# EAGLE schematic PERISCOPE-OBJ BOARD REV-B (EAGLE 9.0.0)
This Set of Many Schematics Is what comprises the Revision-B PCB, of my eden project "PERISCOPE". (OBJECT BOARD ONLY)

## Sheet 1 of 6: Solder Points For Major Signals
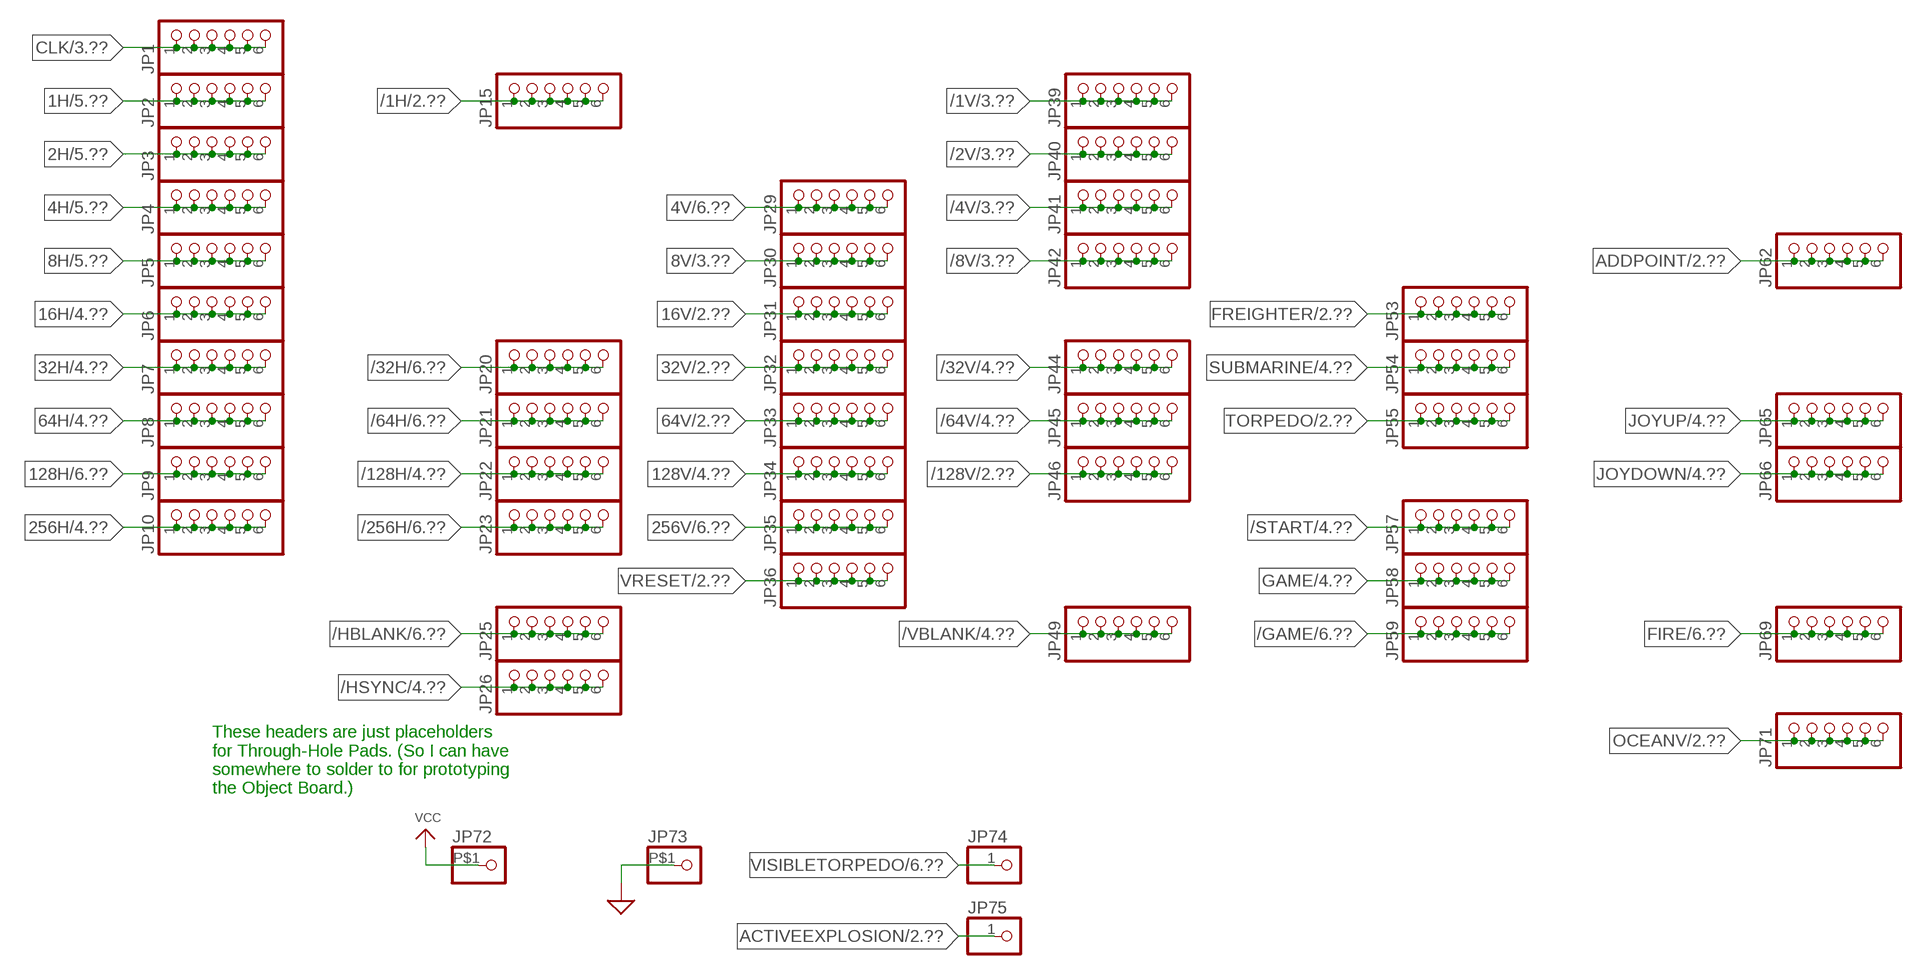
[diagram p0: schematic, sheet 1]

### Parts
JP1  PINHD-1X6  [1X06]
JP2  PINHD-1X6  [1X06]
JP3  PINHD-1X6  [1X06]
JP4  PINHD-1X6  [1X06]
JP5  PINHD-1X6  [1X06]
JP6  PINHD-1X6  [1X06]
JP7  PINHD-1X6  [1X06]
JP8  PINHD-1X6  [1X06]
JP9  PINHD-1X6  [1X06]
JP10  PINHD-1X6  [1X06]
JP15  PINHD-1X6  [1X06]
JP20  PINHD-1X6  [1X06]
JP21  PINHD-1X6  [1X06]
JP22  PINHD-1X6  [1X06]
JP23  PINHD-1X6  [1X06]
JP25  PINHD-1X6  [1X06]
JP26  PINHD-1X6  [1X06]
JP29  PINHD-1X6  [1X06]
JP30  PINHD-1X6  [1X06]
JP31  PINHD-1X6  [1X06]
JP32  PINHD-1X6  [1X06]
JP33  PINHD-1X6  [1X06]
JP34  PINHD-1X6  [1X06]
JP35  PINHD-1X6  [1X06]
JP36  PINHD-1X6  [1X06]
JP39  PINHD-1X6  [1X06]
JP40  PINHD-1X6  [1X06]
JP41  PINHD-1X6  [1X06]
JP42  PINHD-1X6  [1X06]
JP44  PINHD-1X6  [1X06]
JP45  PINHD-1X6  [1X06]
JP46  PINHD-1X6  [1X06]
JP49  PINHD-1X6  [1X06]
JP53  PINHD-1X6  [1X06]
JP54  PINHD-1X6  [1X06]
JP55  PINHD-1X6  [1X06]
JP57  PINHD-1X6  [1X06]
JP58  PINHD-1X6  [1X06]
JP59  PINHD-1X6  [1X06]
JP62  PINHD-1X6  [1X06]
JP65  PINHD-1X6  [1X06]
JP66  PINHD-1X6  [1X06]
JP69  PINHD-1X6  [1X06]
JP71  PINHD-1X6  [1X06]
JP72  PINHD-1X1-BIGPOGO  [1X1-BIGPOGO]
JP73  PINHD-1X1-BIGPOGO  [1X1-BIGPOGO]
JP74  PINHD-1X1  [1X01]
JP75  PINHD-1X1  [1X01]

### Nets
1H: JP2.1 JP2.2 JP2.3 JP2.4 JP2.5 JP2.6 ; also sheet 5
2H: JP3.1 JP3.2 JP3.3 JP3.4 JP3.5 JP3.6 ; also sheet 5
4H: JP4.1 JP4.2 JP4.3 JP4.4 JP4.5 JP4.6 ; also sheet 5
4V: JP29.1 JP29.2 JP29.3 JP29.4 JP29.5 JP29.6 ; also sheet 6
8H: JP5.1 JP5.2 JP5.3 JP5.4 JP5.5 JP5.6 ; also sheet 5,6
8V: JP30.1 JP30.2 JP30.3 JP30.4 JP30.5 JP30.6 ; also sheet 3
16H: JP6.1 JP6.2 JP6.3 JP6.4 JP6.5 JP6.6 ; also sheet 4
16V: JP31.1 JP31.2 JP31.3 JP31.4 JP31.5 JP31.6 ; also sheet 2,4
32H: JP7.1 JP7.2 JP7.3 JP7.4 JP7.5 JP7.6 ; also sheet 4
32V: JP32.1 JP32.2 JP32.3 JP32.4 JP32.5 JP32.6 ; also sheet 2,4
64H: JP8.1 JP8.2 JP8.3 JP8.4 JP8.5 JP8.6 ; also sheet 4
64V: JP33.1 JP33.2 JP33.3 JP33.4 JP33.5 JP33.6 ; also sheet 2,4
128H: JP9.1 JP9.2 JP9.3 JP9.4 JP9.5 JP9.6 ; also sheet 6
128V: JP34.1 JP34.2 JP34.3 JP34.4 JP34.5 JP34.6 ; also sheet 4
256H: JP10.1 JP10.2 JP10.3 JP10.4 JP10.5 JP10.6 ; also sheet 4
256V: JP35.1 JP35.2 JP35.3 JP35.4 JP35.5 JP35.6 ; also sheet 6
/1H: JP15.1 JP15.2 JP15.3 JP15.4 JP15.5 JP15.6 ; also sheet 2
/1V: JP39.1 JP39.2 JP39.3 JP39.4 JP39.5 JP39.6 ; also sheet 3
/2V: JP40.1 JP40.2 JP40.3 JP40.4 JP40.5 JP40.6 ; also sheet 3
/4V: JP41.1 JP41.2 JP41.3 JP41.4 JP41.5 JP41.6 ; also sheet 3
/8V: JP42.1 JP42.2 JP42.3 JP42.4 JP42.5 JP42.6 ; also sheet 3
/32H: JP20.1 JP20.2 JP20.3 JP20.4 JP20.5 JP20.6 ; also sheet 6
/32V: JP44.1 JP44.2 JP44.3 JP44.4 JP44.5 JP44.6 ; also sheet 4
/64H: JP21.1 JP21.2 JP21.3 JP21.4 JP21.5 JP21.6 ; also sheet 6
/64V: JP45.1 JP45.2 JP45.3 JP45.4 JP45.5 JP45.6 ; also sheet 4
/128H: JP22.1 JP22.2 JP22.3 JP22.4 JP22.5 JP22.6 ; also sheet 4
/128V: JP46.1 JP46.2 JP46.3 JP46.4 JP46.5 JP46.6 ; also sheet 2
/256H: JP23.1 JP23.2 JP23.3 JP23.4 JP23.5 JP23.6 ; also sheet 6
/GAME: JP59.1 JP59.2 JP59.3 JP59.4 JP59.5 JP59.6 ; also sheet 6
/HBLANK: JP25.1 JP25.2 JP25.3 JP25.4 JP25.5 JP25.6 ; also sheet 6
/HSYNC: JP26.1 JP26.2 JP26.3 JP26.4 JP26.5 JP26.6 ; also sheet 4,6
/START: JP57.1 JP57.2 JP57.3 JP57.4 JP57.5 JP57.6 ; also sheet 4
/VBLANK: JP49.1 JP49.2 JP49.3 JP49.4 JP49.5 JP49.6 ; also sheet 4,6
ACTIVEEXPLOSION: JP75.1 ; also sheet 2,3
ADDPOINT: JP62.1 JP62.2 JP62.3 JP62.4 JP62.5 JP62.6 ; also sheet 2
CLK: JP1.1 JP1.2 JP1.3 JP1.4 JP1.5 JP1.6 ; also sheet 3,6
FIRE: JP69.1 JP69.2 JP69.3 JP69.4 JP69.5 JP69.6 ; also sheet 6
FREIGHTER: JP53.1 JP53.2 JP53.3 JP53.4 JP53.5 JP53.6 ; also sheet 2
GAME: JP58.1 JP58.2 JP58.3 JP58.4 JP58.5 JP58.6 ; also sheet 4
GND: JP73.P$1 ; supply symbol labelled SUP ; also sheet 2,3,4,5,6
JOYDOWN: JP66.1 JP66.2 JP66.3 JP66.4 JP66.5 JP66.6 ; also sheet 4
JOYUP: JP65.1 JP65.2 JP65.3 JP65.4 JP65.5 JP65.6 ; also sheet 4
OCEANV: JP71.1 JP71.2 JP71.3 JP71.4 JP71.5 JP71.6 ; also sheet 2,6
SUBMARINE: JP54.1 JP54.2 JP54.3 JP54.4 JP54.5 JP54.6 ; also sheet 4
TORPEDO: JP55.1 JP55.2 JP55.3 JP55.4 JP55.5 JP55.6 ; also sheet 2,6
VCC: JP72.P$1 ; also sheet 2,3,4,5,6
VISIBLETORPEDO: JP74.1 ; also sheet 6
VRESET: JP36.1 JP36.2 JP36.3 JP36.4 JP36.5 JP36.6 ; also sheet 2

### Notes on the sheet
- These headers are just placeholders
  for Through-Hole Pads. (So I can have
  somewhere to solder to for prototyping
  the Object Board.)

## Sheet 2 of 6: FREIGHTER MOTION
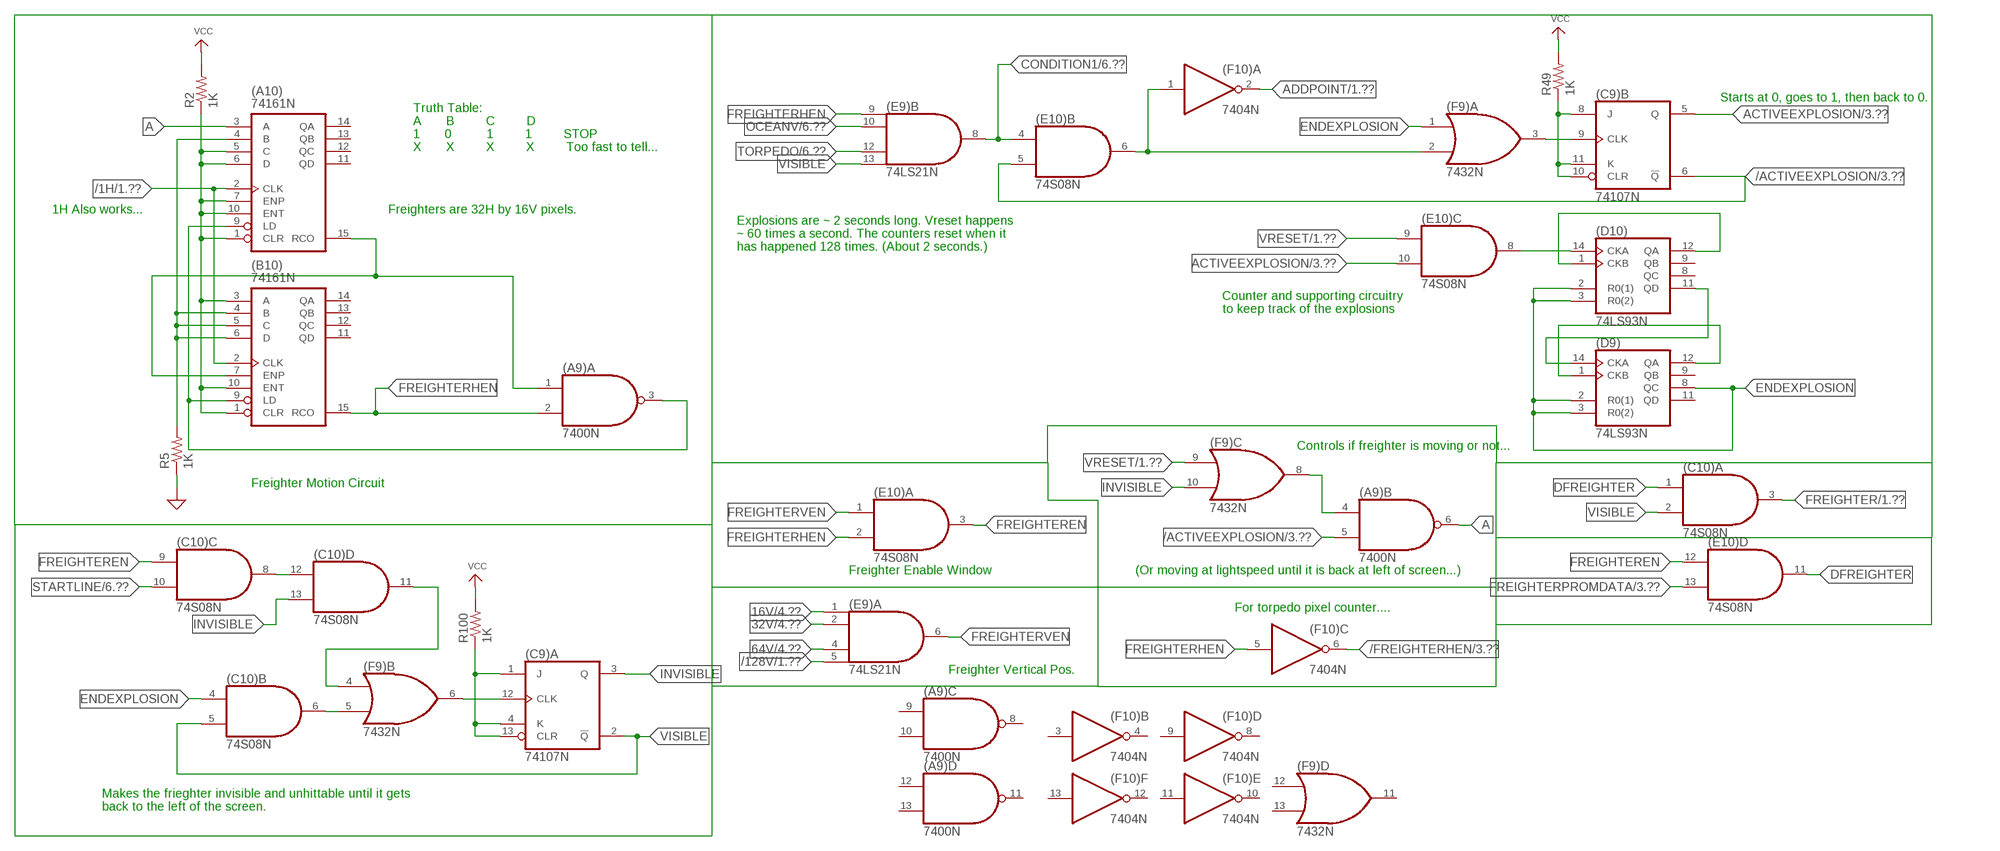
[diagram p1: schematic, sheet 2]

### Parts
(A9)  7400N  [DIL14]
(A10)  74161N  [DIL16]
(B10)  74161N  [DIL16]
(C9)  74107N  [DIL14]
(C10)  74S08N  [DIL14]
(D9)  74LS93N  [DIL14]
(D10)  74LS93N  [DIL14]
(E9)  74LS21N  [DIL14]
(E10)  74S08N  [DIL14]
(F9)  7432N  [DIL14]
(F10)  7404N  [DIL14]
R2  1K  R-US_0207/10  [0207/10]
R5  1K  R-US_0207/10  [0207/10]
R49  1K  R-US_0207/10  [0207/10]
R100  1K  R-US_0207/10  [0207/10]

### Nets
16V: (E9).1(A:I0) ; also sheet 1,4
32V: (E9).2(A:I1) ; also sheet 1,4
64V: (E9).4(A:I2) ; also sheet 1,4
/1H: (A10).2(CLK) (B10).2(CLK) ; also sheet 1
/128V: (E9).5(A:I3) ; also sheet 1
/ACTIVEEXPLOSION: (A9).5(B:I1) (C9).6(B:!Q) (E10).5(B:I1) ; also sheet 3
/FREIGHTERHEN: (F10).6(C:O) ; also sheet 3
A: (A9).6(B:O) (A10).3(A)
ACTIVEEXPLOSION: (C9).5(B:Q) (E10).10(C:I1) ; also sheet 1,3
ADDPOINT: (F10).2(A:O) ; also sheet 1
CONDITION1: (E9).8(B:O) (E10).4(B:I0) ; also sheet 6
DFREIGHTER: (C10).1(A:I0) (E10).11(D:O)
ENDEXPLOSION: (C10).4(B:I0) (D9).2(R0(1)) (D9).3(R0(2)) (D9).8(QC) (D10).2(R0(1)) (D10).3(R0(2)) (F9).1(A:I0)
FREIGHTER: (C10).3(A:O) ; also sheet 1
FREIGHTEREN: (C10).9(C:I0) (E10).3(A:O) (E10).12(D:I0)
FREIGHTERHEN: (A9).2(A:I1) (B10).15(RCO) (E9).9(B:I0) (E10).2(A:I1) (F10).5(C:I)
FREIGHTERPROMDATA: (E10).13(D:I1) ; also sheet 3
FREIGHTERVEN: (E9).6(A:O) (E10).1(A:I0)
GND: R5.1 ; supply symbol labelled SUP ; also sheet 1,3,4,5,6
INVISIBLE: (C9).3(A:Q) (C10).13(D:I1) (F9).10(C:I1)
N$56: (A10).4(B) (B10).4(B) (B10).5(C) (B10).6(D) R5.2
N$57: (A10).1(CLR) (A10).5(C) (A10).6(D) (A10).7(ENP) (A10).10(ENT) (B10).1(CLR) (B10).3(A) (B10).10(ENT) R2.1
N$59: (D10).1(CKB) (D10).12(QA)
N$60: (A9).3(A:O) (A10).9(LD) (B10).9(LD)
N$62: (D9).1(CKB) (D9).12(QA)
N$63: (A9).1(A:I0) (A10).15(RCO) (B10).7(ENP)
N$64: (D10).14(CKA) (E10).8(C:O)
N$67: (D9).14(CKA) (D10).11(QD)
N$68: (C9).9(B:CLK) (F9).3(A:O)
N$69: (C9).8(B:J) (C9).10(B:CLR) (C9).11(B:K) R49.1
N$71: (E10).6(B:O) (F9).2(A:I1) (F10).1(A:I)
N$116: (C9).12(A:CLK) (F9).6(B:O)
N$141: (C10).6(B:O) (F9).5(B:I1)
N$142: (C9).1(A:J) (C9).4(A:K) (C9).13(A:CLR) R100.1
N$143: (C10).8(C:O) (C10).12(D:I0)
N$165: (C10).11(D:O) (F9).4(B:I0)
N$166: (A9).4(B:I0) (F9).8(C:O)
OCEANV: (E9).10(B:I1) ; also sheet 1,6
STARTLINE: (C10).10(C:I1) ; also sheet 6
TORPEDO: (E9).12(B:I2) ; also sheet 1,6
VCC: R2.2 R49.2 R100.2 ; also sheet 1,3,4,5,6
VISIBLE: (C9).2(A:!Q) (C10).2(A:I1) (C10).5(B:I1) (E9).13(B:I3)
VRESET: (E10).9(C:I0) (F9).9(C:I0) ; also sheet 1
Unconnected: (A9).8(C:O) (A9).9(C:I0) (A9).10(C:I1) (A9).11(D:O) (A9).12(D:I0) (A9).13(D:I1) (A10).11(QD) (A10).12(QC) (A10).13(QB) (A10).14(QA) (B10).11(QD) (B10).12(QC) (B10).13(QB) (B10).14(QA) (D9).9(QB) (D9).11(QD) (D10).8(QC) (D10).9(QB) (F9).11(D:O) (F9).12(D:I0) (F9).13(D:I1) (F10).3(B:I) (F10).4(B:O) (F10).8(D:O) (F10).9(D:I) (F10).10(E:O) (F10).11(E:I) (F10).12(F:O) (F10).13(F:I)

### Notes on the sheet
- Starts at 0, goes to 1, then back to 0.
- Truth Table:
  A       B         C         D
  1       0          1         1         STOP
  X       X         X         X         Too fast to tell...
- 1H Also works... | Freighters are 32H by 16V pixels.
- Explosions are ~ 2 seconds long. Vreset happens
  ~ 60 times a second. The counters reset when it
  has happened 128 times. (About 2 seconds.)
- Counter and supporting circuitry
  to keep track of the explosions
- Controls if freighter is moving or not...
- Freighter Motion Circuit
- Freighter Enable Window | (Or moving at lightspeed until it is back at left of screen...)
- For torpedo pixel counter....
- Freighter Vertical Pos.
- Makes the frieghter invisible and unhittable until it gets
  back to the left of the screen.

## Sheet 3 of 6: FREIGHTER GRAPHICS
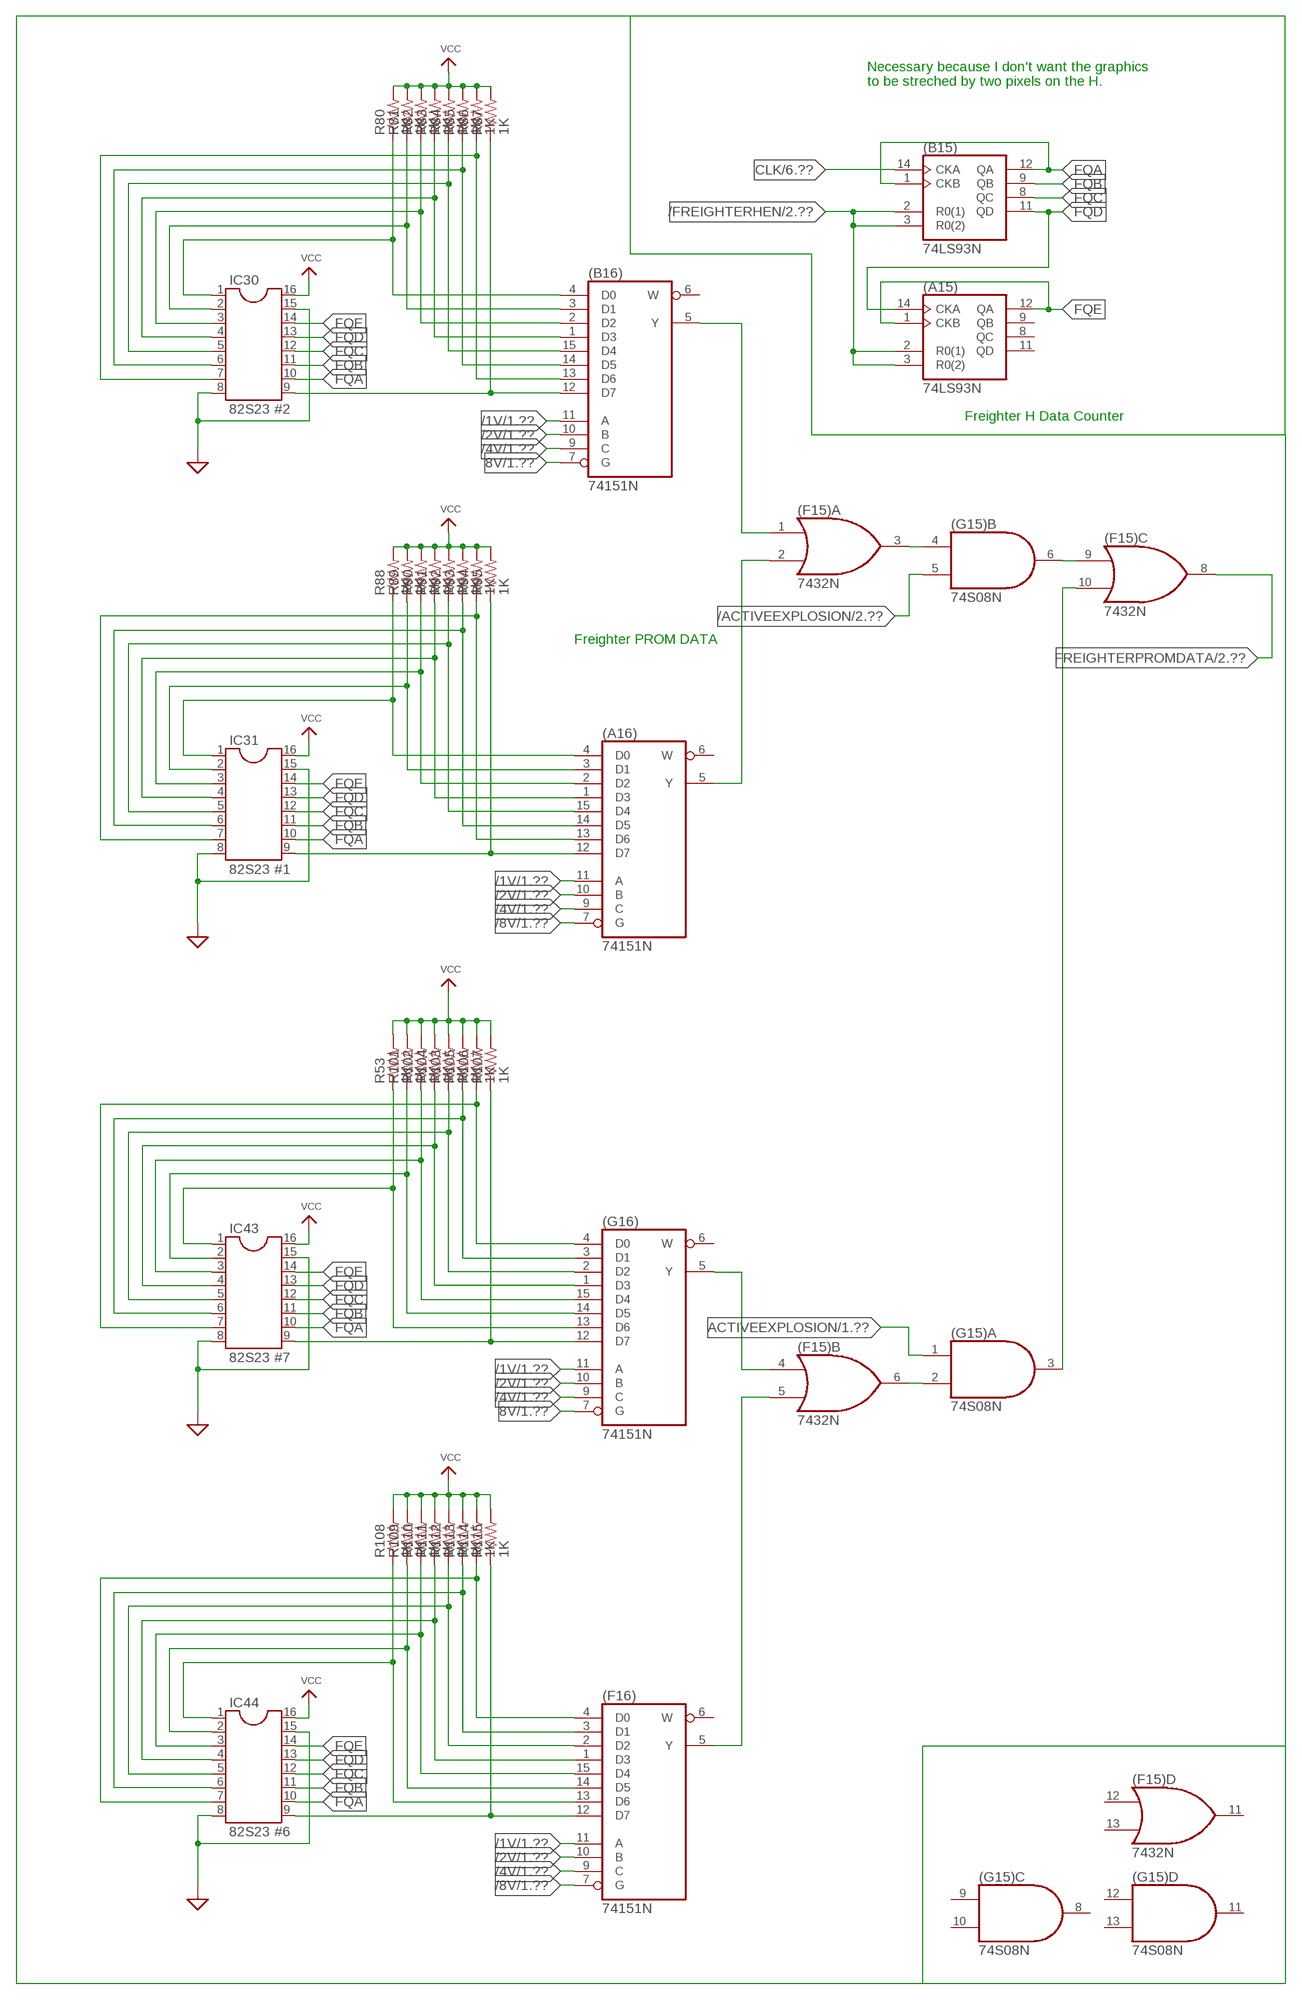
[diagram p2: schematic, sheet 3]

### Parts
(A15)  74LS93N  [DIL14]
(A16)  74151N  [DIL16]
(B15)  74LS93N  [DIL14]
(B16)  74151N  [DIL16]
(F15)  7432N  [DIL14]
(F16)  74151N  [DIL16]
(G15)  74S08N  [DIL14]
(G16)  74151N  [DIL16]
IC30  82S23 #2  DIL16S  [SOCKET-16]
IC31  82S23 #1  DIL16S  [SOCKET-16]
IC43  82S23 #7  DIL16S  [SOCKET-16]
IC44  82S23 #6  DIL16S  [SOCKET-16]
R53  1K  R-US_0207/10  [0207/10]
R80  1K  R-US_0207/10  [0207/10]
R81  1K  R-US_0207/10  [0207/10]
R82  1K  R-US_0207/10  [0207/10]
R83  1K  R-US_0207/10  [0207/10]
R84  1K  R-US_0207/10  [0207/10]
R85  1K  R-US_0207/10  [0207/10]
R86  1K  R-US_0207/10  [0207/10]
R87  1K  R-US_0207/10  [0207/10]
R88  1K  R-US_0207/10  [0207/10]
R89  1K  R-US_0207/10  [0207/10]
R90  1K  R-US_0207/10  [0207/10]
R91  1K  R-US_0207/10  [0207/10]
R92  1K  R-US_0207/10  [0207/10]
R93  1K  R-US_0207/10  [0207/10]
R94  1K  R-US_0207/10  [0207/10]
R95  1K  R-US_0207/10  [0207/10]
R101  1K  R-US_0207/10  [0207/10]
R102  1K  R-US_0207/10  [0207/10]
R103  1K  R-US_0207/10  [0207/10]
R104  1K  R-US_0207/10  [0207/10]
R105  1K  R-US_0207/10  [0207/10]
R106  1K  R-US_0207/10  [0207/10]
R107  1K  R-US_0207/10  [0207/10]
R108  1K  R-US_0207/10  [0207/10]
R109  1K  R-US_0207/10  [0207/10]
R110  1K  R-US_0207/10  [0207/10]
R111  1K  R-US_0207/10  [0207/10]
R112  1K  R-US_0207/10  [0207/10]
R113  1K  R-US_0207/10  [0207/10]
R114  1K  R-US_0207/10  [0207/10]
R115  1K  R-US_0207/10  [0207/10]

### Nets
8V: (B16).7(G) (G16).7(G) ; also sheet 1
/1V: (A16).11(A) (B16).11(A) (F16).11(A) (G16).11(A) ; also sheet 1
/2V: (A16).10(B) (B16).10(B) (F16).10(B) (G16).10(B) ; also sheet 1
/4V: (A16).9(C) (B16).9(C) (F16).9(C) (G16).9(C) ; also sheet 1
/8V: (A16).7(G) (F16).7(G) ; also sheet 1
/ACTIVEEXPLOSION: (G15).5(B:I1) ; also sheet 2
/FREIGHTERHEN: (A15).2(R0(1)) (A15).3(R0(2)) (B15).2(R0(1)) (B15).3(R0(2)) ; also sheet 2
ACTIVEEXPLOSION: (G15).1(A:I0) ; also sheet 1,2
CLK: (B15).14(CKA) ; also sheet 1,6
FQA: (B15).1(CKB) (B15).12(QA) IC30.10 IC31.10 IC43.10 IC44.10
FQB: (B15).9(QB) IC30.11 IC31.11 IC43.11 IC44.11
FQC: (B15).8(QC) IC30.12 IC31.12 IC43.12 IC44.12
FQD: (A15).14(CKA) (B15).11(QD) IC30.13 IC31.13 IC43.13 IC44.13
FQE: (A15).1(CKB) (A15).12(QA) IC30.14 IC31.14 IC43.14 IC44.14
FREIGHTERPROMDATA: (F15).8(C:O) ; also sheet 2
GND: IC30.8 IC30.15 IC31.8 IC31.15 IC43.8 IC43.15 IC44.8 IC44.15 ; supply symbol labelled SUP ; also sheet 1,2,4,5,6
N$58: (F15).3(A:O) (G15).4(B:I0)
N$98: (A16).4(D0) IC31.1 R88.1
N$100: (A16).3(D1) IC31.2 R89.1
N$103: (A16).2(D2) IC31.3 R90.1
N$104: (A16).1(D3) IC31.4 R91.1
N$106: (A16).15(D4) IC31.5 R92.1
N$108: (A16).14(D5) IC31.6 R93.1
N$110: (A16).13(D6) IC31.7 R94.1
N$111: (A16).12(D7) IC31.9 R95.1
N$120: (B16).12(D7) IC30.9 R87.1
N$121: (B16).13(D6) IC30.7 R86.1
N$122: (B16).14(D5) IC30.6 R85.1
N$123: (B16).15(D4) IC30.5 R84.1
N$124: (B16).1(D3) IC30.4 R83.1
N$125: (B16).2(D2) IC30.3 R82.1
N$126: (B16).3(D1) IC30.2 R81.1
N$127: (B16).4(D0) IC30.1 R80.1
N$134: (B16).5(Y) (F15).1(A:I0)
N$135: (A16).5(Y) (F15).2(A:I1)
N$144: (F16).12(D7) IC44.9 R115.1
N$145: (F15).4(B:I0) (G16).5(Y)
N$146: (F15).5(B:I1) (F16).5(Y)
N$147: (F15).9(C:I0) (G15).6(B:O)
N$148: (F15).10(C:I1) (G15).3(A:O)
N$149: (F15).6(B:O) (G15).2(A:I1)
N$150: (G16).12(D7) IC43.9 R107.1
N$151: (G16).13(D6) IC43.1 R53.1
N$152: (G16).14(D5) IC43.2 R101.1
N$153: (G16).15(D4) IC43.3 R102.1
N$154: (G16).1(D3) IC43.4 R104.1
N$155: (G16).2(D2) IC43.5 R103.1
N$156: (G16).3(D1) IC43.6 R105.1
N$157: (G16).4(D0) IC43.7 R106.1
N$158: (F16).13(D6) IC44.1 R108.1
N$159: (F16).14(D5) IC44.2 R109.1
N$160: (F16).15(D4) IC44.3 R110.1
N$161: (F16).1(D3) IC44.4 R111.1
N$162: (F16).2(D2) IC44.5 R112.1
N$163: (F16).3(D1) IC44.6 R113.1
N$164: (F16).4(D0) IC44.7 R114.1
VCC: IC30.16 IC31.16 IC43.16 IC44.16 R53.2 R80.2 R81.2 R82.2 R83.2 R84.2 R85.2 R86.2 R87.2 R88.2 R89.2 R90.2 R91.2 R92.2 R93.2 R94.2 R95.2 R101.2 R102.2 R103.2 R104.2 R105.2 R106.2 R107.2 R108.2 R109.2 R110.2 R111.2 R112.2 R113.2 R114.2 R115.2 ; also sheet 1,2,4,5,6
Unconnected: (A15).8(QC) (A15).9(QB) (A15).11(QD) (A16).6(W) (B16).6(W) (F15).11(D:O) (F15).12(D:I0) (F15).13(D:I1) (F16).6(W) (G15).8(C:O) (G15).9(C:I0) (G15).10(C:I1) (G15).11(D:O) (G15).12(D:I0) (G15).13(D:I1) (G16).6(W)

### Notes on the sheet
- Necessary because I don't want the graphics
  to be streched by two pixels on the H.
- Freighter H Data Counter
- Freighter PROM DATA

## Sheet 4 of 6: SUBMARINE MOTION
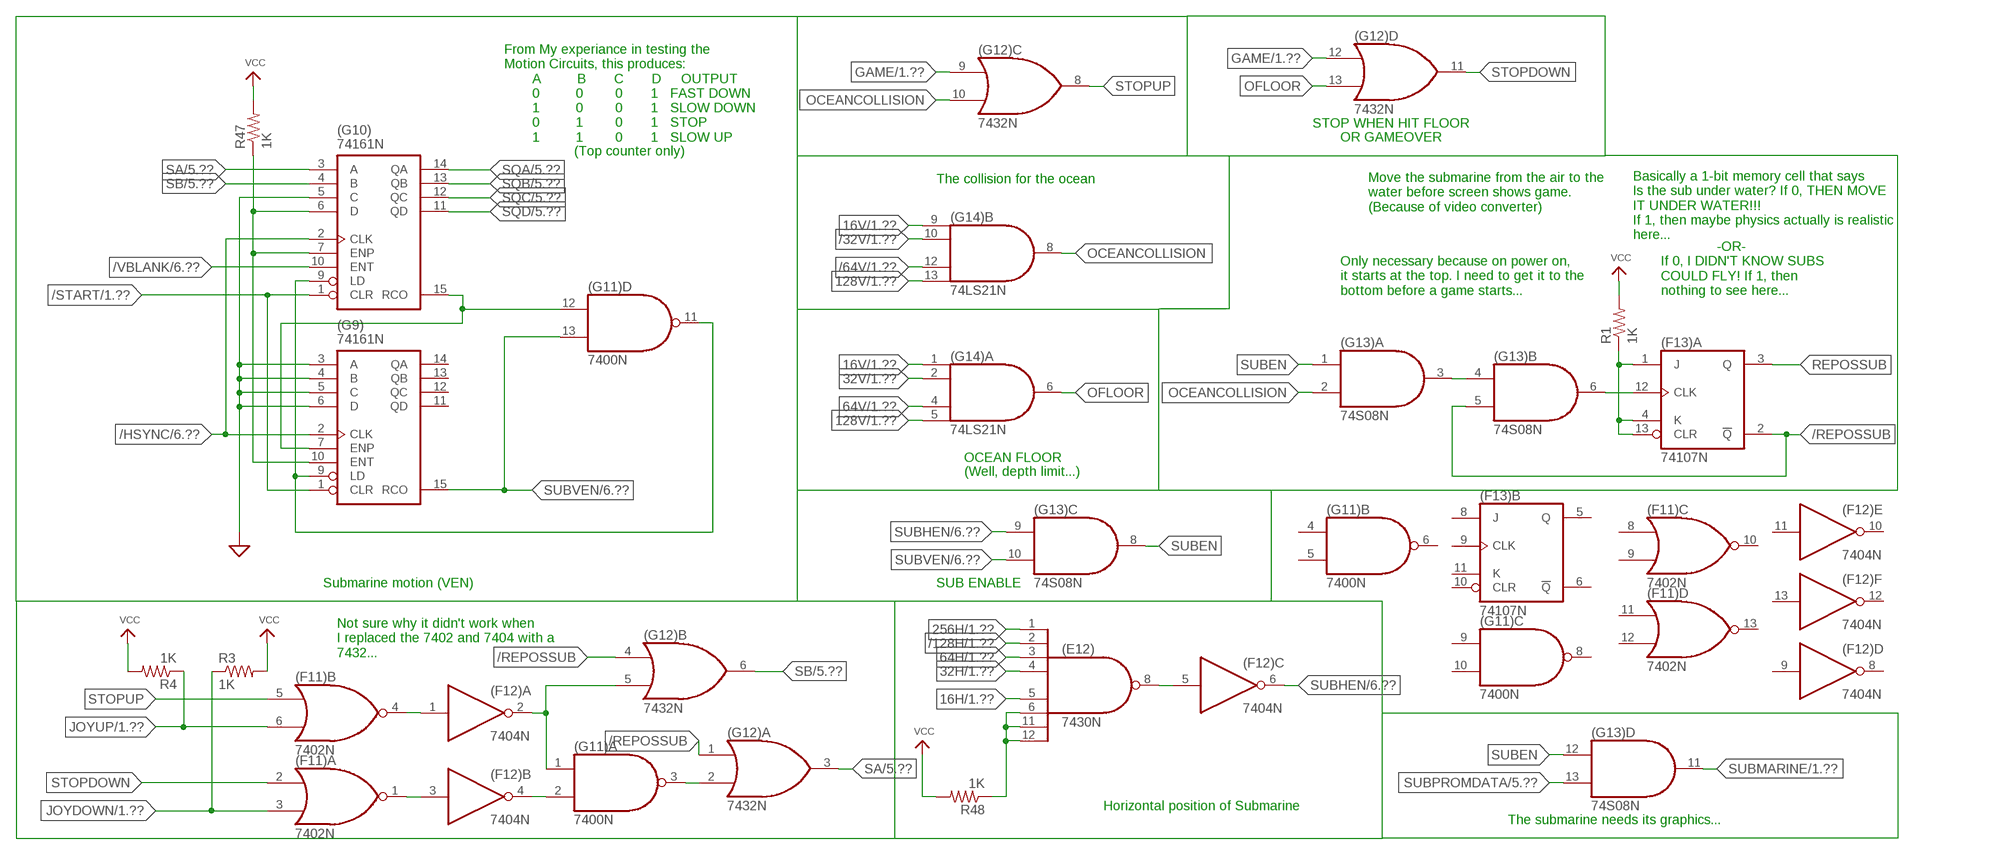
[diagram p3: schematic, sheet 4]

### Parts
(E12)  7430N  [DIL14]
(F11)  7402N  [DIL14]
(F12)  7404N  [DIL14]
(F13)  74107N  [DIL14]
(G9)  74161N  [DIL16]
(G10)  74161N  [DIL16]
(G11)  7400N  [DIL14]
(G12)  7432N  [DIL14]
(G13)  74S08N  [DIL14]
(G14)  74LS21N  [DIL14]
R1  1K  R-US_0207/10  [0207/10]
R3  1K  R-US_0207/10  [0207/10]
R4  1K  R-US_0207/10  [0207/10]
R47  1K  R-US_0207/10  [0207/10]
R48  1K  R-US_0207/10  [0207/10]

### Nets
16H: (E12).5(I4) ; also sheet 1
16V: (G14).1(A:I0) (G14).9(B:I0) ; also sheet 1,2
32H: (E12).4(I3) ; also sheet 1
32V: (G14).2(A:I1) ; also sheet 1,2
64H: (E12).3(I2) ; also sheet 1
64V: (G14).4(A:I2) ; also sheet 1,2
128V: (G14).5(A:I3) (G14).13(B:I3) ; also sheet 1
256H: (E12).1(I0) ; also sheet 1
/32V: (G14).10(B:I1) ; also sheet 1
/64V: (G14).12(B:I2) ; also sheet 1
/128H: (E12).2(I1) ; also sheet 1
/HSYNC: (G9).2(CLK) (G10).2(CLK) ; also sheet 1,6
/REPOSSUB: (F13).2(A:!Q) (G12).1(A:I0) (G12).4(B:I0) (G13).5(B:I1)
/START: (G9).1(CLR) (G10).1(CLR) ; also sheet 1
/VBLANK: (G10).10(ENT) ; also sheet 1,6
BB: (F12).2(A:O) (G11).1(A:I0) (G12).5(B:I1)
GAME: (G12).9(C:I0) (G12).12(D:I0) ; also sheet 1
GND: (G9).3(A) (G9).4(B) (G9).5(C) (G9).6(D) (G10).5(C) ; supply symbol labelled SUP ; also sheet 1,2,3,5,6
JOYDOWN: (F11).3(A:I1) R3.1 ; also sheet 1
JOYUP: (F11).6(B:I1) R4.1 ; also sheet 1
N$1: (F11).1(A:O) (F12).3(B:I)
N$9: (F12).4(B:O) (G11).2(A:I1)
N$41: (F11).4(B:O) (F12).1(A:I)
N$48: (E12).8(O) (F12).5(C:I)
N$50: (G9).10(ENT) (G10).6(D) (G10).7(ENP) R47.1
N$51: (G9).9(LD) (G10).9(LD) (G11).11(D:O)
N$52: (E12).6(I5) (E12).11(I6) (E12).12(I7) R48.1
N$53: (F13).1(A:J) (F13).4(A:K) (F13).13(A:CLR) R1.1
N$54: (G13).3(A:O) (G13).4(B:I0)
N$55: (F13).12(A:CLK) (G13).6(B:O)
N$170: (G11).3(A:O) (G12).2(A:I1)
N$173: (G9).7(ENP) (G10).15(RCO) (G11).12(D:I0)
OCEANCOLLISION: (G12).10(C:I1) (G13).2(A:I1) (G14).8(B:O)
OFLOOR: (G12).13(D:I1) (G14).6(A:O)
REPOSSUB: (F13).3(A:Q)
SA: (G10).3(A) (G12).3(A:O) ; also sheet 5,6
SB: (G10).4(B) (G12).6(B:O) ; also sheet 5,6
SQA: (G10).14(QA) ; also sheet 5
SQB: (G10).13(QB) ; also sheet 5,6
SQC: (G10).12(QC) ; also sheet 5
SQD: (G10).11(QD) ; also sheet 5,6
STOPDOWN: (F11).2(A:I0) (G12).11(D:O)
STOPUP: (F11).5(B:I0) (G12).8(C:O)
SUBEN: (G13).1(A:I0) (G13).8(C:O) (G13).12(D:I0)
SUBHEN: (F12).6(C:O) (G13).9(C:I0) ; also sheet 6
SUBMARINE: (G13).11(D:O) ; also sheet 1
SUBPROMDATA: (G13).13(D:I1) ; also sheet 5
SUBVEN: (G9).15(RCO) (G11).13(D:I1) (G13).10(C:I1) ; also sheet 6
VCC: R1.2 R3.2 R4.2 R47.2 R48.2 ; also sheet 1,2,3,5,6
Unconnected: (F11).8(C:I0) (F11).9(C:I1) (F11).10(C:O) (F11).11(D:I0) (F11).12(D:I1) (F11).13(D:O) (F12).8(D:O) (F12).9(D:I) (F12).10(E:O) (F12).11(E:I) (F12).12(F:O) (F12).13(F:I) (F13).5(B:Q) (F13).6(B:!Q) (F13).8(B:J) (F13).9(B:CLK) (F13).10(B:CLR) (F13).11(B:K) (G9).11(QD) (G9).12(QC) (G9).13(QB) (G9).14(QA) (G11).4(B:I0) (G11).5(B:I1) (G11).6(B:O) (G11).8(C:O) (G11).9(C:I0) (G11).10(C:I1)

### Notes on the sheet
- STOP WHEN HIT FLOOR
- From My experiance in testing the 
  Motion Circuits, this produces:
         A         B       C       D     OUTPUT
         0         0        0       1   FAST DOWN
         1         0        0       1   SLOW DOWN
         0         1        0       1   STOP
         1         1        0       1   SLOW UP
- OR GAMEOVER
- (Top counter only)
- The collision for the ocean
- Move the submarine from the air to the
  water before screen shows game. 
  (Because of video converter)
- Basically a 1-bit memory cell that says
  Is the sub under water? If 0, THEN MOVE
  IT UNDER WATER!!!
  If 1, then maybe physics actually is realistic
  here...
- Only necessary because on power on,
  it starts at the top. I need to get it to the
  bottom before a game starts...
- -OR-
  If 0, I DIDN'T KNOW SUBS
  COULD FLY! If 1, then 
  nothing to see here...
- OCEAN FLOOR
- (Well, depth limit...)
- Submarine motion (VEN) | SUB ENABLE
- Not sure why it didn't work when
  I replaced the 7402 and 7404 with a
  7432...
- Horizontal position of Submarine
- The submarine needs its graphics...

## Sheet 5 of 6: SUBMARINE GRAPHICS
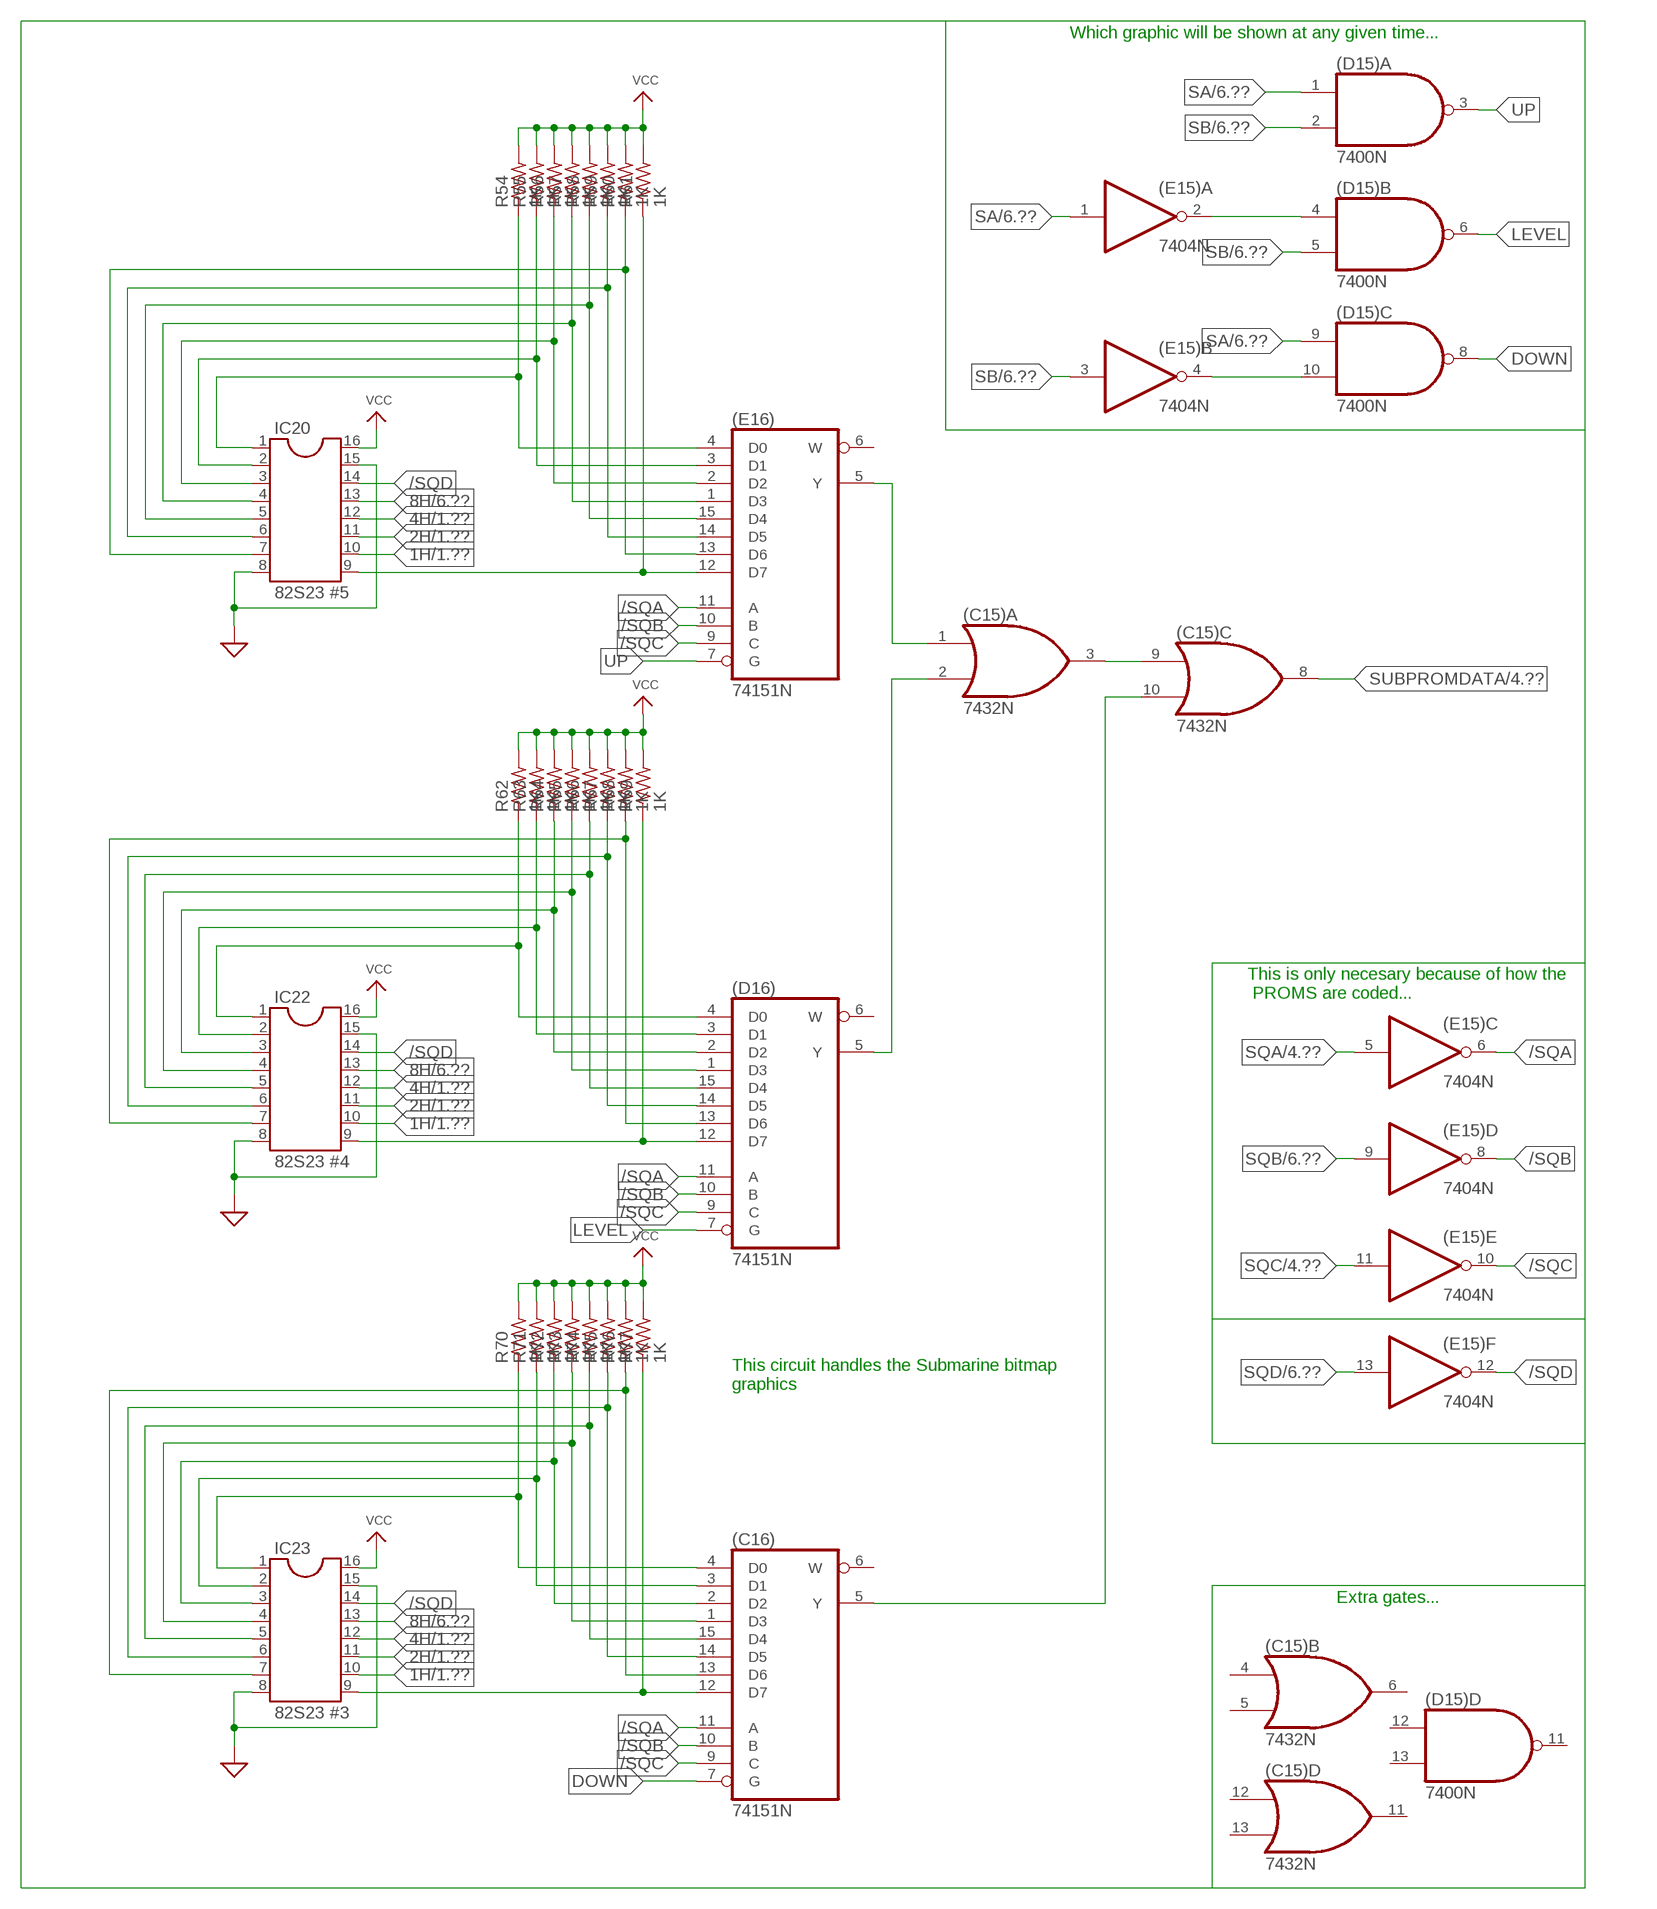
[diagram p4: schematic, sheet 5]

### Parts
(C15)  7432N  [DIL14]
(C16)  74151N  [DIL16]
(D15)  7400N  [DIL14]
(D16)  74151N  [DIL16]
(E15)  7404N  [DIL14]
(E16)  74151N  [DIL16]
IC20  82S23 #5  DIL16S  [SOCKET-16]
IC22  82S23 #4  DIL16S  [SOCKET-16]
IC23  82S23 #3  DIL16S  [SOCKET-16]
R54  1K  R-US_0207/10  [0207/10]
R55  1K  R-US_0207/10  [0207/10]
R56  1K  R-US_0207/10  [0207/10]
R57  1K  R-US_0207/10  [0207/10]
R58  1K  R-US_0207/10  [0207/10]
R59  1K  R-US_0207/10  [0207/10]
R60  1K  R-US_0207/10  [0207/10]
R61  1K  R-US_0207/10  [0207/10]
R62  1K  R-US_0207/10  [0207/10]
R63  1K  R-US_0207/10  [0207/10]
R64  1K  R-US_0207/10  [0207/10]
R65  1K  R-US_0207/10  [0207/10]
R66  1K  R-US_0207/10  [0207/10]
R67  1K  R-US_0207/10  [0207/10]
R68  1K  R-US_0207/10  [0207/10]
R69  1K  R-US_0207/10  [0207/10]
R70  1K  R-US_0207/10  [0207/10]
R71  1K  R-US_0207/10  [0207/10]
R72  1K  R-US_0207/10  [0207/10]
R73  1K  R-US_0207/10  [0207/10]
R74  1K  R-US_0207/10  [0207/10]
R75  1K  R-US_0207/10  [0207/10]
R76  1K  R-US_0207/10  [0207/10]
R77  1K  R-US_0207/10  [0207/10]

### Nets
1H: IC20.10 IC22.10 IC23.10 ; also sheet 1
2H: IC20.11 IC22.11 IC23.11 ; also sheet 1
4H: IC20.12 IC22.12 IC23.12 ; also sheet 1
8H: IC20.13 IC22.13 IC23.13 ; also sheet 1,6
/SQA: (C16).11(A) (D16).11(A) (E15).6(C:O) (E16).11(A)
/SQB: (C16).10(B) (D16).10(B) (E15).8(D:O) (E16).10(B)
/SQC: (C16).9(C) (D16).9(C) (E15).10(E:O) (E16).9(C)
/SQD: (E15).12(F:O) IC20.14 IC22.14 IC23.14
DOWN: (C16).7(G) (D15).8(C:O)
GND: IC20.8 IC20.15 IC22.8 IC22.15 IC23.8 IC23.15 ; supply symbol labelled SUP ; also sheet 1,2,3,4,6
LEVEL: (D15).6(B:O) (D16).7(G)
N$65: (C15).1(A:I0) (E16).5(Y)
N$66: (C15).2(A:I1) (D16).5(Y)
N$72: (C15).10(C:I1) (C16).5(Y)
N$73: (E16).12(D7) IC20.9 R61.1
N$74: (E16).1(D3) IC20.4 R57.1
N$75: (E16).15(D4) IC20.5 R58.1
N$76: (C15).3(A:O) (C15).9(C:I0)
N$77: (E16).14(D5) IC20.6 R59.1
N$78: (E16).13(D6) IC20.7 R60.1
N$79: (C16).4(D0) IC23.1 R70.1
N$80: (D16).4(D0) IC22.1 R62.1
N$81: (D16).3(D1) IC22.2 R63.1
N$82: (D16).12(D7) IC22.9 R69.1
N$83: (C16).12(D7) IC23.9 R77.1
N$84: (E16).4(D0) IC20.1 R54.1
N$85: (E16).3(D1) IC20.2 R55.1
N$86: (E16).2(D2) IC20.3 R56.1
N$87: (D16).2(D2) IC22.3 R64.1
N$88: (D16).1(D3) IC22.4 R65.1
N$89: (D16).15(D4) IC22.5 R66.1
N$90: (D16).14(D5) IC22.6 R67.1
N$91: (D16).13(D6) IC22.7 R68.1
N$92: (C16).3(D1) IC23.2 R71.1
N$93: (C16).2(D2) IC23.3 R72.1
N$94: (C16).1(D3) IC23.4 R73.1
N$95: (C16).15(D4) IC23.5 R74.1
N$96: (C16).14(D5) IC23.6 R75.1
N$97: (C16).13(D6) IC23.7 R76.1
N$102: (D15).10(C:I1) (E15).4(B:O)
N$105: (D15).4(B:I0) (E15).2(A:O)
SA: (D15).1(A:I0) (D15).9(C:I0) (E15).1(A:I) ; also sheet 4,6
SB: (D15).2(A:I1) (D15).5(B:I1) (E15).3(B:I) ; also sheet 4,6
SQA: (E15).5(C:I) ; also sheet 4
SQB: (E15).9(D:I) ; also sheet 4,6
SQC: (E15).11(E:I) ; also sheet 4
SQD: (E15).13(F:I) ; also sheet 4,6
SUBPROMDATA: (C15).8(C:O) ; also sheet 4
UP: (D15).3(A:O) (E16).7(G)
VCC: IC20.16 IC22.16 IC23.16 R54.2 R55.2 R56.2 R57.2 R58.2 R59.2 R60.2 R61.2 R62.2 R63.2 R64.2 R65.2 R66.2 R67.2 R68.2 R69.2 R70.2 R71.2 R72.2 R73.2 R74.2 R75.2 R76.2 R77.2 ; also sheet 1,2,3,4,6
Unconnected: (C15).4(B:I0) (C15).5(B:I1) (C15).6(B:O) (C15).11(D:O) (C15).12(D:I0) (C15).13(D:I1) (C16).6(W) (D15).11(D:O) (D15).12(D:I0) (D15).13(D:I1) (D16).6(W) (E16).6(W)

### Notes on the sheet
- Which graphic will be shown at any given time...
- This is only necesary because of how the
   PROMS are coded...
- This circuit handles the Submarine bitmap
  graphics
- Extra gates...

## Sheet 6 of 6: TORPEDO MOTION
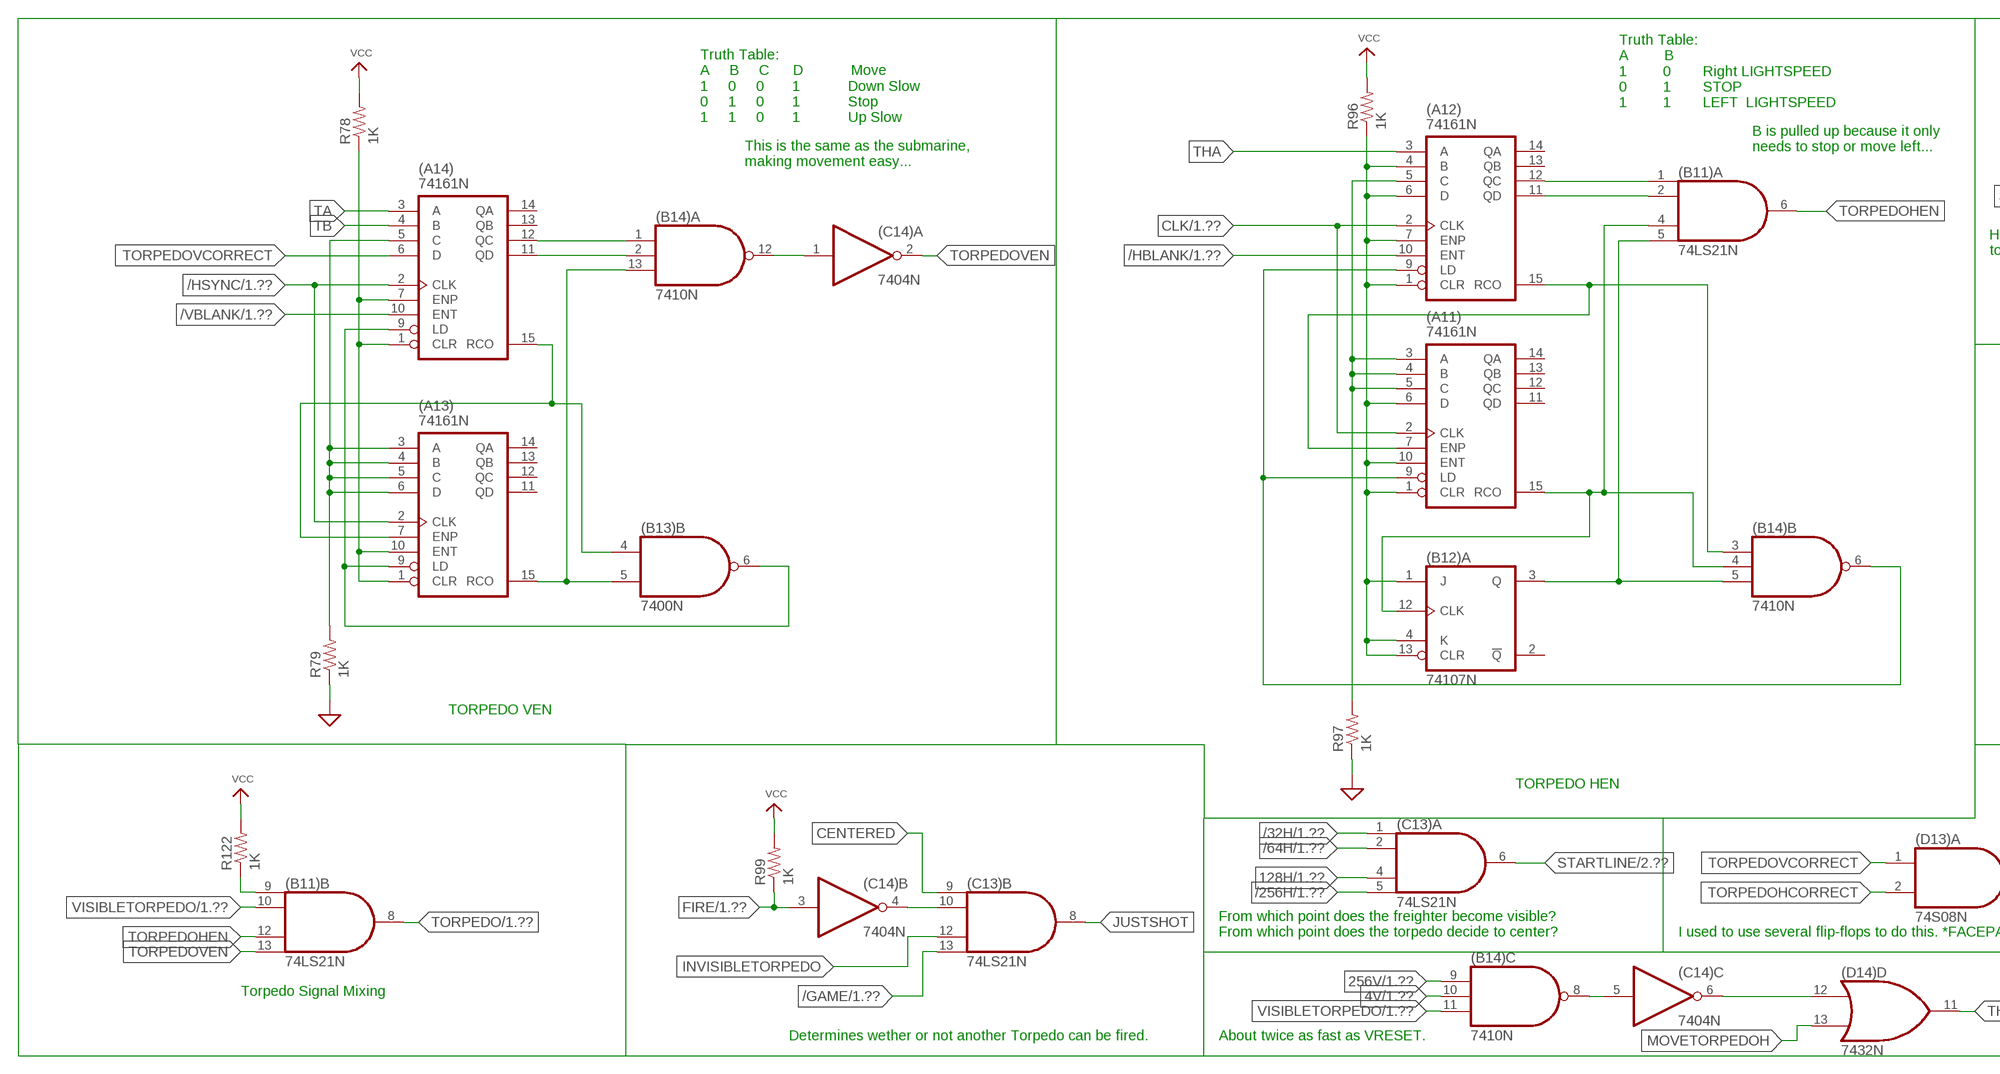
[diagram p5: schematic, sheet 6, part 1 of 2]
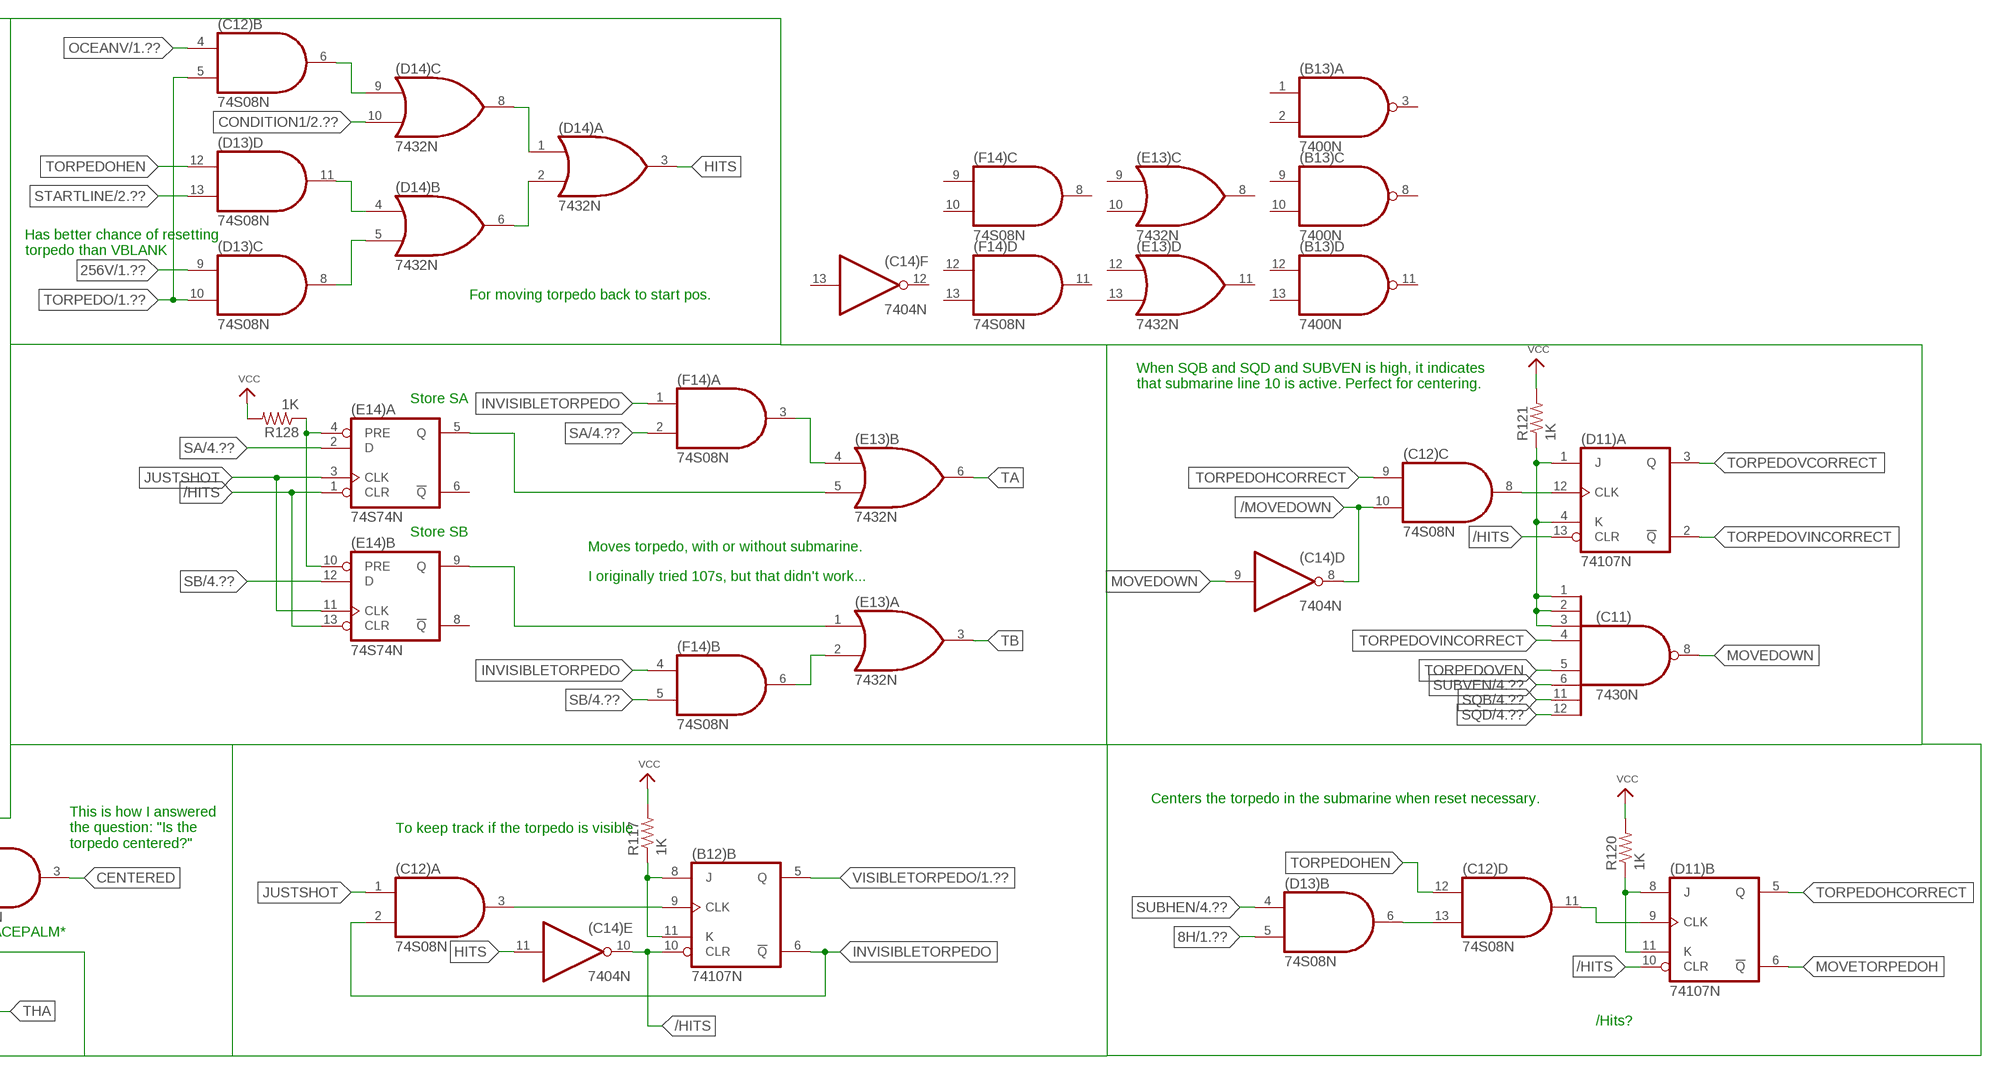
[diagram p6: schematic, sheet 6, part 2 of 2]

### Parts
(A11)  74161N  [DIL16]
(A12)  74161N  [DIL16]
(A13)  74161N  [DIL16]
(A14)  74161N  [DIL16]
(B11)  74LS21N  [DIL14]
(B12)  74107N  [DIL14]
(B13)  7400N  [DIL14]
(B14)  7410N  [DIL14]
(C11)  7430N  [DIL14]
(C12)  74S08N  [DIL14]
(C13)  74LS21N  [DIL14]
(C14)  7404N  [DIL14]
(D11)  74107N  [DIL14]
(D13)  74S08N  [DIL14]
(D14)  7432N  [DIL14]
(E13)  7432N  [DIL14]
(E14)  74S74N  [DIL14]
(F14)  74S08N  [DIL14]
R78  1K  R-US_0207/10  [0207/10]
R79  1K  R-US_0207/10  [0207/10]
R96  1K  R-US_0207/10  [0207/10]
R97  1K  R-US_0207/10  [0207/10]
R99  1K  R-US_0207/10  [0207/10]
R117  1K  R-US_0207/10  [0207/10]
R120  1K  R-US_0207/10  [0207/10]
R121  1K  R-US_0207/10  [0207/10]
R122  1K  R-US_0207/10  [0207/10]
R128  1K  R-US_0207/10  [0207/10]

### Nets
4V: (B14).10(C:I1) ; also sheet 1
8H: (D13).5(B:I1) ; also sheet 1,5
128H: (C13).4(A:I2) ; also sheet 1
256V: (B14).9(C:I0) (D13).9(C:I0) ; also sheet 1
/32H: (C13).1(A:I0) ; also sheet 1
/64H: (C13).2(A:I1) ; also sheet 1
/256H: (C13).5(A:I3) ; also sheet 1
/GAME: (C13).13(B:I3) ; also sheet 1
/HBLANK: (A12).10(ENT) ; also sheet 1
/HITS: (B12).10(B:CLR) (C14).10(E:O) (D11).10(B:CLR) (D11).13(A:CLR) (E14).1(A:CLR) (E14).13(B:CLR)
/HSYNC: (A13).2(CLK) (A14).2(CLK) ; also sheet 1,4
/MOVEDOWN: (C12).10(C:I1) (C14).8(D:O)
/VBLANK: (A14).10(ENT) ; also sheet 1,4
CENTERED: (C13).9(B:I0) (D13).3(A:O)
CLK: (A11).2(CLK) (A12).2(CLK) ; also sheet 1,3
CONDITION1: (D14).10(C:I1) ; also sheet 2
FIRE: (C14).3(B:I) R99.1 ; also sheet 1
GND: R79.1 R97.1 ; supply symbol labelled SUP ; also sheet 1,2,3,4,5
HITS: (C14).11(E:I) (D14).3(A:O)
INVISIBLETORPEDO: (B12).6(B:!Q) (C12).2(A:I1) (C13).12(B:I2) (F14).1(A:I0) (F14).4(B:I0)
JUSTSHOT: (C12).1(A:I0) (C13).8(B:O) (E14).3(A:CLK) (E14).11(B:CLK)
MOVEDOWN: (C11).8(O) (C14).9(D:I)
MOVETORPEDOH: (D11).6(B:!Q) (D14).13(D:I1)
N$49: (C12).8(C:O) (D11).12(A:CLK)
N$61: (A13).3(A) (A13).4(B) (A13).5(C) (A13).6(D) (A14).5(C) R79.2
N$107: (A12).12(QC) (B11).1(A:I0)
N$109: (A12).11(QD) (B11).2(A:I1)
N$112: (A11).3(A) (A11).4(B) (A11).5(C) (A12).5(C) R97.2
N$113: (C13).10(B:I1) (C14).4(B:O)
N$115: (B11).5(A:I3) (B12).3(A:Q) (B14).5(B:I2)
N$119: (A11).9(LD) (A12).9(LD) (B14).6(B:O)
N$128: (A13).1(CLR) (A13).10(ENT) (A14).1(CLR) (A14).7(ENP) R78.1
N$129: (C12).13(D:I1) (D13).6(B:O)
N$130: (A13).9(LD) (A14).9(LD) (B13).6(B:O)
N$131: (A13).15(RCO) (B13).5(B:I1) (B14).13(A:I2)
N$132: (A13).7(ENP) (A14).15(RCO) (B13).4(B:I0)
N$133: (A14).12(QC) (B14).1(A:I0)
N$136: (A14).11(QD) (B14).2(A:I1)
N$137: (A11).7(ENP) (A12).15(RCO) (B14).3(B:I0)
N$138: (B14).12(A:O) (C14).1(A:I)
N$139: (A11).15(RCO) (B11).4(A:I2) (B12).12(A:CLK) (B14).4(B:I1)
N$140: (A11).1(CLR) (A11).6(D) (A11).10(ENT) (A12).1(CLR) (A12).4(B) (A12).6(D) (A12).7(ENP) (B12).1(A:J) (B12).4(A:K) (B12).13(A:CLR) R96.1
N$167: (B14).8(C:O) (C14).5(C:I)
N$168: (C14).6(C:O) (D14).12(D:I0)
N$171: (C12).6(B:O) (D14).9(C:I0)
N$172: (C12).11(D:O) (D11).9(B:CLK)
N$174: (D14).2(A:I1) (D14).6(B:O)
N$175: (B12).8(B:J) (B12).11(B:K) R117.1
N$176: (D13).11(D:O) (D14).4(B:I0)
N$177: (D13).8(C:O) (D14).5(B:I1)
N$179: (D14).1(A:I0) (D14).8(C:O)
N$187: (D11).8(B:J) (D11).11(B:K) R120.1
N$190: (B12).9(B:CLK) (C12).3(A:O)
N$191: (B11).9(B:I0) R122.1
N$192: (C11).1(I0) (C11).2(I1) (C11).3(I2) (D11).1(A:J) (D11).4(A:K) R121.1
N$200: (E14).4(A:PRE) (E14).10(B:PRE) R128.1
N$201: (E13).5(B:I1) (E14).5(A:Q)
N$210: (E13).1(A:I0) (E14).9(B:Q)
N$212: (E13).4(B:I0) (F14).3(A:O)
N$213: (E13).2(A:I1) (F14).6(B:O)
OCEANV: (C12).4(B:I0) ; also sheet 1,2
SA: (E14).2(A:D) (F14).2(A:I1) ; also sheet 4,5
SB: (E14).12(B:D) (F14).5(B:I1) ; also sheet 4,5
SQB: (C11).11(I6) ; also sheet 4,5
SQD: (C11).12(I7) ; also sheet 4,5
STARTLINE: (C13).6(A:O) (D13).13(D:I1) ; also sheet 2
SUBHEN: (D13).4(B:I0) ; also sheet 4
SUBVEN: (C11).6(I5) ; also sheet 4
TA: (A14).3(A) (E13).6(B:O)
TB: (A14).4(B) (E13).3(A:O)
THA: (A12).3(A) (D14).11(D:O)
TORPEDO: (B11).8(B:O) (C12).5(B:I1) (D13).10(C:I1) ; also sheet 1,2
TORPEDOHCORRECT: (C12).9(C:I0) (D11).5(B:Q) (D13).2(A:I1)
TORPEDOHEN: (B11).6(A:O) (B11).12(B:I2) (C12).12(D:I0) (D13).12(D:I0)
TORPEDOVCORRECT: (A14).6(D) (D11).3(A:Q) (D13).1(A:I0)
TORPEDOVEN: (B11).13(B:I3) (C11).5(I4) (C14).2(A:O)
TORPEDOVINCORRECT: (C11).4(I3) (D11).2(A:!Q)
VCC: R78.2 R96.2 R99.2 R117.2 R120.2 R121.2 R122.2 R128.2 ; also sheet 1,2,3,4,5
VISIBLETORPEDO: (B11).10(B:I1) (B12).5(B:Q) (B14).11(C:I2) ; also sheet 1
Unconnected: (A11).11(QD) (A11).12(QC) (A11).13(QB) (A11).14(QA) (A12).13(QB) (A12).14(QA) (A13).11(QD) (A13).12(QC) (A13).13(QB) (A13).14(QA) (A14).13(QB) (A14).14(QA) (B12).2(A:!Q) (B13).1(A:I0) (B13).2(A:I1) (B13).3(A:O) (B13).8(C:O) (B13).9(C:I0) (B13).10(C:I1) (B13).11(D:O) (B13).12(D:I0) (B13).13(D:I1) (C14).12(F:O) (C14).13(F:I) (E13).8(C:O) (E13).9(C:I0) (E13).10(C:I1) (E13).11(D:O) (E13).12(D:I0) (E13).13(D:I1) (E14).6(A:!Q) (E14).8(B:!Q) (F14).8(C:O) (F14).9(C:I0) (F14).10(C:I1) (F14).11(D:O) (F14).12(D:I0) (F14).13(D:I1)

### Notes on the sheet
- Truth Table:
  A         B    
  1         0        Right LIGHTSPEED
  0         1        STOP
  1         1        LEFT  LIGHTSPEED
- Truth Table:
  A     B     C      D            Move
  1     0     0       1            Down Slow
  0     1     0       1            Stop
  1     1     0       1            Up Slow
- B is pulled up because it only
  needs to stop or move left...
- This is the same as the submarine,
  making movement easy...
- Has better chance of resetting 
  torpedo than VBLANK
- For moving torpedo back to start pos.
- When SQB and SQD and SUBVEN is high, it indicates
  that submarine line 10 is active. Perfect for centering.
- Store SA
- Store SB
- Moves torpedo, with or without submarine.
- I originally tried 107s, but that didn't work...
- TORPEDO VEN
- TORPEDO HEN
- Centers the torpedo in the submarine when reset necessary.
- To keep track if the torpedo is visible
- This is how I answered
  the question: "Is the 
  torpedo centered?"
- From which point does the freighter become visible?
  From which point does the torpedo decide to center?
- I used to use several flip-flops to do this. *FACEPALM*
- Torpedo Signal Mixing
- /Hits?
- Determines wether or not another Torpedo can be fired. | About twice as fast as VRESET.

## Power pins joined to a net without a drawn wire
GND: (A9).7(P:GND) (A10).8(GND) (A11).8(GND) (A12).8(GND) (A13).8(GND) (A14).8(GND) (A15).10(GND) (A16).8(GND) (B10).8(GND) (B11).7(P:GND) (B12).7(P:GND) (B13).7(P:GND) (B14).7(P:GND) (B15).10(GND) (B16).8(GND) (C9).7(P:GND) (C10).7(P:GND) (C11).7(GND) (C12).7(P:GND) (C13).7(P:GND) (C14).7(P:GND) (C15).7(P:GND) (C16).8(GND) (D9).10(GND) (D10).10(GND) (D11).7(P:GND) (D13).7(P:GND) (D14).7(P:GND) (D15).7(P:GND) (D16).8(GND) (E9).7(P:GND) (E10).7(P:GND) (E12).7(GND) (E13).7(P:GND) (E14).7(P:GND) (E15).7(P:GND) (E16).8(GND) (F9).7(P:GND) (F10).7(P:GND) (F11).7(P:GND) (F12).7(P:GND) (F13).7(P:GND) (F14).7(P:GND) (F15).7(P:GND) (F16).8(GND) (G9).8(GND) (G10).8(GND) (G11).7(P:GND) (G12).7(P:GND) (G13).7(P:GND) (G14).7(P:GND) (G15).7(P:GND) (G16).8(GND)
VCC: (A9).14(P:VCC) (A10).16(VCC) (A11).16(VCC) (A12).16(VCC) (A13).16(VCC) (A14).16(VCC) (A15).5(VCC) (A16).16(VCC) (B10).16(VCC) (B11).14(P:VCC) (B12).14(P:VCC) (B13).14(P:VCC) (B14).14(P:VCC) (B15).5(VCC) (B16).16(VCC) (C9).14(P:VCC) (C10).14(P:VCC) (C11).14(VCC) (C12).14(P:VCC) (C13).14(P:VCC) (C14).14(P:VCC) (C15).14(P:VCC) (C16).16(VCC) (D9).5(VCC) (D10).5(VCC) (D11).14(P:VCC) (D13).14(P:VCC) (D14).14(P:VCC) (D15).14(P:VCC) (D16).16(VCC) (E9).14(P:VCC) (E10).14(P:VCC) (E12).14(VCC) (E13).14(P:VCC) (E14).14(P:VCC) (E15).14(P:VCC) (E16).16(VCC) (F9).14(P:VCC) (F10).14(P:VCC) (F11).14(P:VCC) (F12).14(P:VCC) (F13).14(P:VCC) (F14).14(P:VCC) (F15).14(P:VCC) (F16).16(VCC) (G9).16(VCC) (G10).16(VCC) (G11).14(P:VCC) (G12).14(P:VCC) (G13).14(P:VCC) (G14).14(P:VCC) (G15).14(P:VCC) (G16).16(VCC)

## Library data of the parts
(A9) (B13) (D15) (G11) = 74xx-us:74*00: Quad 2-input NAND gate
(A10) (A11) (A12) (A13) (A14) (B10) (G9) (G10) = oldchips:74*161: Synchronous 4-bit COUNTER with direct clear
(A15) (B15) (D9) (D10) = 74xx-us:74*93: Decade, divide by twelve and binary COUNTER
(A16) (B16) (C16) (D16) (E16) (F16) (G16) = 74xx-us:74*151: Data SELECTOR/MULTIPLEXER
(B11) (C13) (E9) (G14) = 74xx-us:74*21: Dual 4-input AND gate
(B12) (C9) (D11) (F13) = 74xx-us:74*107: Dual J-K FLIP FLOP, clear
(B14) = 74xx-us:74*10: Triple 3-input NAND gate
(C10) (C12) (D13) (E10) (F14) (G13) (G15) = 74xx-us:74*08: Quad 2-input AND gate
(C11) (E12) = 74xx-us:74*30: 8-input NAND gate
(C14) (E15) (F10) (F12) = 74xx-us:74*04: Hex INVERTER
(C15) (D14) (E13) (F9) (F15) (G12) = 74xx-us:74*32: Quad 2-input OR gate
(E14) = 74xx-us:74*74: Dual D type positive edge triggered FLIP FLOP, preset and clear
(F11) = 74xx-us:74*02: Quad 2-input NOR gate
IC20 IC22 IC23 IC30 IC31 IC43 IC44 = ic-package:DIL16: Dual In Line / Socket
JP1-JP10 JP15 JP20-JP23 JP25 JP26 JP29-JP36 JP39-JP42 JP44-JP46 JP49 JP53-JP55 JP57-JP59 JP62 JP65 JP66 JP69 JP71 = adafruit:PINHD-1X6: PIN HEADER
JP72-JP75 = adafruit:PINHD-1X1: Pin header 1x1 for 0.1" spacing
R1-R5 R47-R49 R53-R97 R99-R115 R117 R120-R122 R128 = adafruit:R-US_: RESISTOR, American symbol

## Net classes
0 default: width 0.508 mm, clearance 0.254 mm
